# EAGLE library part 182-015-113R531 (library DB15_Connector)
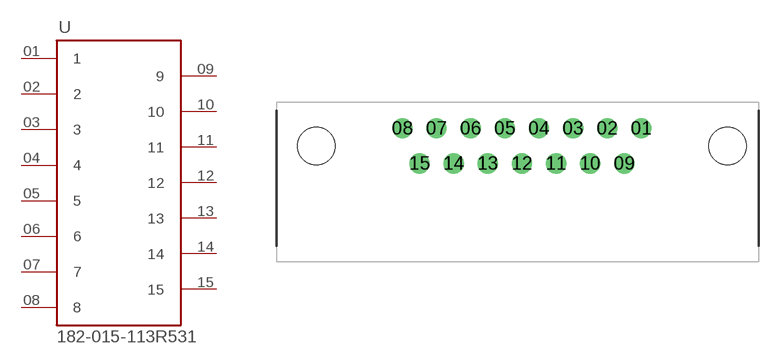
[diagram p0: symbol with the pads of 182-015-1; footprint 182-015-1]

Designator prefix -

## 182-015-113R5311-3R531  [182-015-1]
01  1
02  2
03  3
04  4
05  5
06  6
07  7
08  8
09  9
10  10
11  11
12  12
13  13
14  14
15  15

## Footprint 182-015-1 (pad centres in mm)
drill 1.092 pad 1.524: 01 9.69,1.422; 02 6.921,1.422; 03 4.153,1.422; 04 1.384,1.422; 05 -1.384,1.422; 06 -4.153,1.422; 07 -6.921,1.422; 08 -9.69,1.422; 09 8.306,-1.422; 10 5.537,-1.422; 11 2.769,-1.422; 12 0,-1.422; 13 -2.769,-1.422; 14 -5.537,-1.422; 15 -8.306,-1.422
hole 3.048 at -16.662,0
hole 3.048 at 16.662,0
